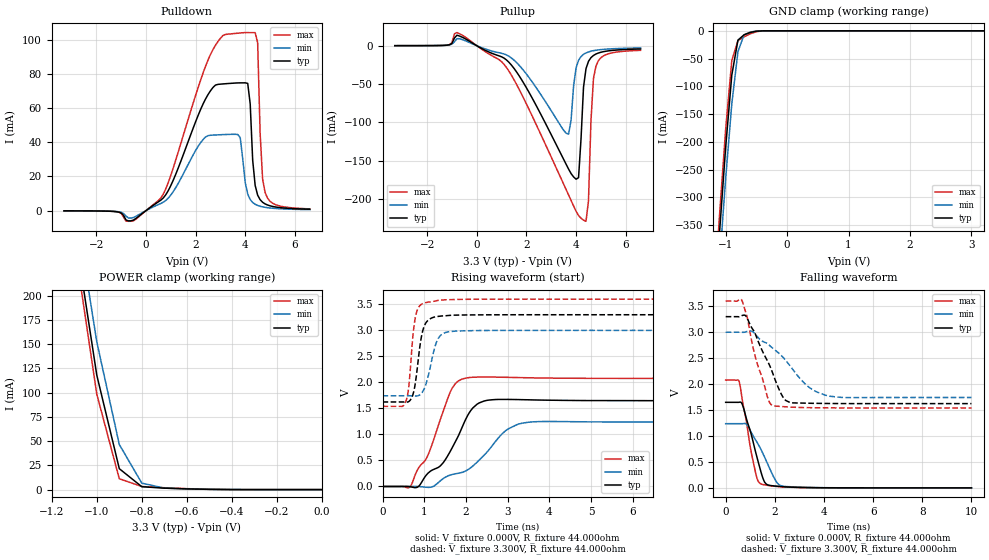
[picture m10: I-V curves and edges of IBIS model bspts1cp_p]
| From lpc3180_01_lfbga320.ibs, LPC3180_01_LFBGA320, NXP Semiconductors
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| |   Rev 0.20 IBIS Model Design Automation Generation   |
| |   N O N - S I L I C O N   C O R R E L A T E D   |
| |   This IBIS [Model] is pre-Beta tactical support   |
| |  Note: this IBIS [Model] contains clamp curves generated   |
| |   through simulation which should not be relied upon   |
| bspts1cp
|   Bidirectional Pad 3v3
|   3state Output
|   Plain Input
|   1ns Slew Rate control
|   CMOS
|   Programmable between
|   - (p1=0, p2=1) plain input
|   - (p1=0, p2=0) with Pull Up
|   - (p1=1, p2=1) with Pull Down
|   - (p1=1, p2=0) with Repeater
|   Characterized at Core 1.2V and I/O 3.3V
| Plain input Mode (p1=0, p2=1)
[Model]   bspts1cp_p | of bspts1cp
Model_type   I/O
Polarity   Non-Inverting
Enable   Active-Low
|  Reciever Thresholds
Vinl   = 0.36V
Vinh   = 0.84V
| AC Test Load Conditions
Vref   = 0
Cref   = 1.2e-11
Rref   = 1000000000
Vmeas   = 0.6
| [Process Range]   typical   min   max
| C_comp edge width   400.000ps   400.000ps   400.000ps
| C_comp Tstrobe   40.000fs   40.000fs   40.000fs
C_comp   2.380pF   2.241pF   2.550pF
[Temperature Range]   25   125   -40
[Voltage Range]   3.30V   3.00V   3.60V
[GND Clamp Reference]   0.00V   0.00V   0.00V
[Pulldown Reference]   0.00V   0.00V   0.00V
[POWER Clamp Reference]   3.30V   3.00V   3.60V
[Pullup Reference]   3.30V   3.00V   3.60V
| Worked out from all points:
|   slope of the pulldown table from 0 to 0.495 V, typ, clamps not added: 97.1 ohm
|   slope of the pullup table from 0 to 0.495 V, typ, clamps not added: 59.3 ohm
|   GND clamp passes 1 mA (typ) near -0.51 V on its own axis
|   POWER clamp passes 1 mA (typ) near -0.63 V on its own axis
|   rising waveform, V_fixture 0.000V, R_fixture 44.000ohm: 20-80 % time 780ps typ, 1.07ns min, 629ps max; typ from 0 V to 1.65 V
|   falling waveform, V_fixture 0.000V, R_fixture 44.000ohm: 20-80 % time 570ps typ, 781ps min, 473ps max; typ from 1.65 V to 0 V
|   rising waveform, V_fixture 3.300V, R_fixture 44.000ohm: 20-80 % time 175ps typ, 231ps min, 140ps max; typ from 1.62 V to 3.3 V
|   falling waveform, V_fixture 3.300V, R_fixture 44.000ohm: 20-80 % time 909ps typ, 1.48ns min, 670ps max; typ from 3.3 V to 1.62 V
[GND Clamp]
| ref voltage   0.00V   0.00V   0.00V
|   Voltage   I(typ)   I(min)   I(max)
-3.3V     -4.198A    -4.223A    -4.188A
-1.2V     -526mA     -577.5mA   -497.2mA
-1.1V     -363.6mA   -417.9mA   -332.6mA
-1V       -210.1mA   -266.3mA   -177.3mA
-900mV    -79.7mA    -131.5mA   -53.27mA
-800mV    -16.73mA   -37.37mA   -17.76mA
-700mV    -7.134mA   -7.247mA   -10.88mA
-600mV    -2.975mA   -2.186mA   -5.408mA
-500mV    -676.3uA   -558.4uA   -1.581mA
-400mV    -60.83uA   -85.23uA   -138.3uA
3.2V      712.7pA    549nA      572.1pA
[Power Clamp]   | Vtable = Vcc - Vpad
| ref voltage   3.30V   3.00V   3.60V
|   Voltage   I(typ)   I(min)   I(max)
-3.3V     4.52A      4.504A     4.537A
-1.1V     269.9mA    299.6mA    255.2mA
-1V       118.1mA    152.4mA    98.45mA
-900mV    21.58mA    46.51mA    11.18mA
-800mV    2.986mA    6.648mA    3.206mA
-700mV    1.495mA    1.532mA    1.933mA
-600mV    740.8uA    686.7uA    976.4uA
-400mV    40.41uA    69.77uA    40.29uA
0V        755.1pA    5.591nA    627.9pA
[Pulldown]
| ref voltage   0.00V   0.00V   0.00V
|   Voltage   I(typ)   I(min)   I(max)
-3.3V     -80.68uA   -69.9uA    -74.32uA
-600mV    -5.92mA    -4.329mA   -6.173mA
500mV     5.147mA    3.568mA    5.923mA
2.5V      67.8mA     43.83mA    87.99mA
3.7V      74.65mA    44.53mA    103.7mA
4V        74.69mA    16.44mA    104.1mA
4.2V      62.37mA    6.514mA    104mA
4.3V      29.48mA    4.769mA    104mA
4.5V      9.068mA    3.068mA    98.16mA
4.6V      6.413mA    2.587mA    45.13mA
4.8V      3.956mA    1.96mA     10.6mA
6.6V      844.8uA    597.5uA    1.056mA
[Pullup]   | Vtable = Vcc - Vpad
| ref voltage   3.30V   3.00V   3.60V
|   Voltage   I(typ)   I(min)   I(max)
-3.3V     39.4uA     37.84uA    38.83uA
-800mV    13.66mA    9.122mA    17.15mA
1V        -14.52mA   -9.936mA   -20.86mA
3.7V      -161.3mA   -115.5mA   -195.1mA
4V        -174.4mA   -29.02mA   -216.2mA
4.1V      -172.4mA   -19.17mA   -221.9mA
4.4V      -30.01mA   -9.422mA   -229.4mA
4.5V      -20.39mA   -8.135mA   -202.5mA
4.6V      -15.6mA    -7.195mA   -97.89mA
4.7V      -12.75mA   -6.48mA    -42.98mA
4.8V      -10.87mA   -5.92mA    -26.67mA
6.6V      -4.278mA   -2.929mA   -6.056mA
[Ramp]
R_load   = 44.000ohm
|   dV/dt(typ)   dV/dt(min)   dV/dt(max)
dV/dt_r   1.003V/795.000ps   754.701mV/1.100ns   1.261V/635.000ps
dV/dt_f   1.022V/900.000ps   769.371mV/1.445ns   1.253V/655.000ps
[Rising Waveform]  | cubic spline decimation from 2001 points
V_fixture   = 0.000V
R_fixture   = 44.000ohm
|   Time   V(typ)   V(min)   V(max)
0s        20.67nV    394.6nV    10.71nV
655ps     -4.49mV    426.4uV    -8.705mV
1.09ns    255.7mV    -17.2mV    604.2mV
1.445ns   447.9mV    146.5mV    1.426V
1.67ns    745.2mV    230.8mV    1.891V
1.975ns   1.26V      292.1mV    2.079V
2.43ns    1.641V     598.3mV    2.104V
2.935ns   1.673V     1.062V     2.098V
3.48ns    1.666V     1.233V     2.089V
10ns      1.649V     1.237V     2.077V
[Falling Waveform]  | cubic spline decimation from 2001 points
V_fixture   = 0.000V
R_fixture   = 44.000ohm
|   Time   V(typ)   V(min)   V(max)
0s        1.649V     1.237V     2.077V
550ps     1.651V     1.237V     2.046V
715ps     1.559V     1.239V     1.589V
1.2ns     725.7mV    936.5mV    330.5mV
1.305ns   535.6mV    855.2mV    145.2mV
1.445ns   292.8mV    731.1mV    74.37mV
1.665ns   69.58mV    507.7mV    51.03mV
2.075ns   32.25mV    108.5mV    27.47mV
2.34ns    22.08mV    31.87mV    18.43mV
10ns      530.2nV    1.313uV    542.6nV
[Rising Waveform]  | cubic spline decimation from 2001 points
V_fixture   = 3.300V
V_fixture_min = 3.000V
V_fixture_max = 3.600V
R_fixture   = 44.000ohm
|   Time   V(typ)   V(min)   V(max)
0s        1.624V     1.742V     1.54V
555ps     1.622V     1.743V     1.63V
625ps     1.63V      1.743V     1.891V
730ps     1.77V      1.741V     2.905V
785ps     1.981V     1.739V     3.244V
920ps     2.823V     1.777V     3.494V
1.005ns   3.092V     1.89V      3.527V
1.31ns    3.265V     2.805V     3.572V
1.585ns   3.286V     2.972V     3.589V
10ns      3.3V       3V         3.6V
[Falling Waveform]  | cubic spline decimation from 2001 points
V_fixture   = 3.300V
V_fixture_min = 3.000V
V_fixture_max = 3.600V
R_fixture   = 44.000ohm
|   Time   V(typ)   V(min)   V(max)
0s        3.3V       3V         3.6V
670ps     3.322V     2.999V     3.604V
840ps     3.3V       3.01V      3.345V
1.255ns   2.908V     2.934V     2.442V
1.735ns   2.414V     2.767V     1.702V
1.9ns     2.229V     2.698V     1.588V
2.44ns    1.686V     2.46V      1.562V
3.24ns    1.633V     2V         1.547V
4.065ns   1.627V     1.785V     1.542V
10ns      1.624V     1.742V     1.54V
